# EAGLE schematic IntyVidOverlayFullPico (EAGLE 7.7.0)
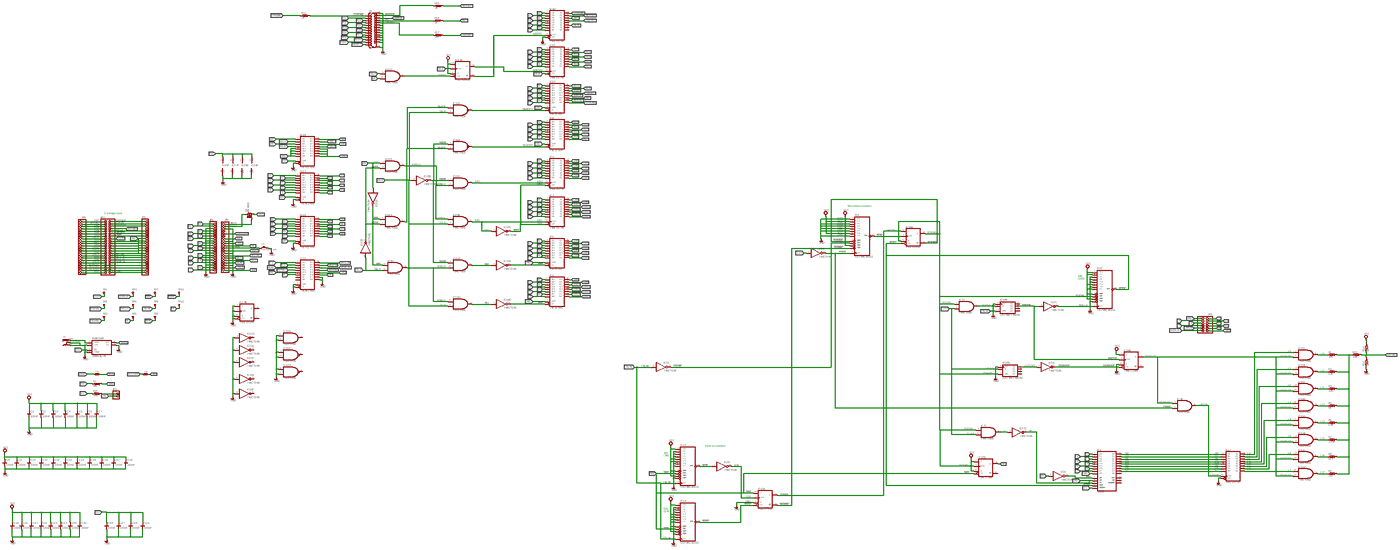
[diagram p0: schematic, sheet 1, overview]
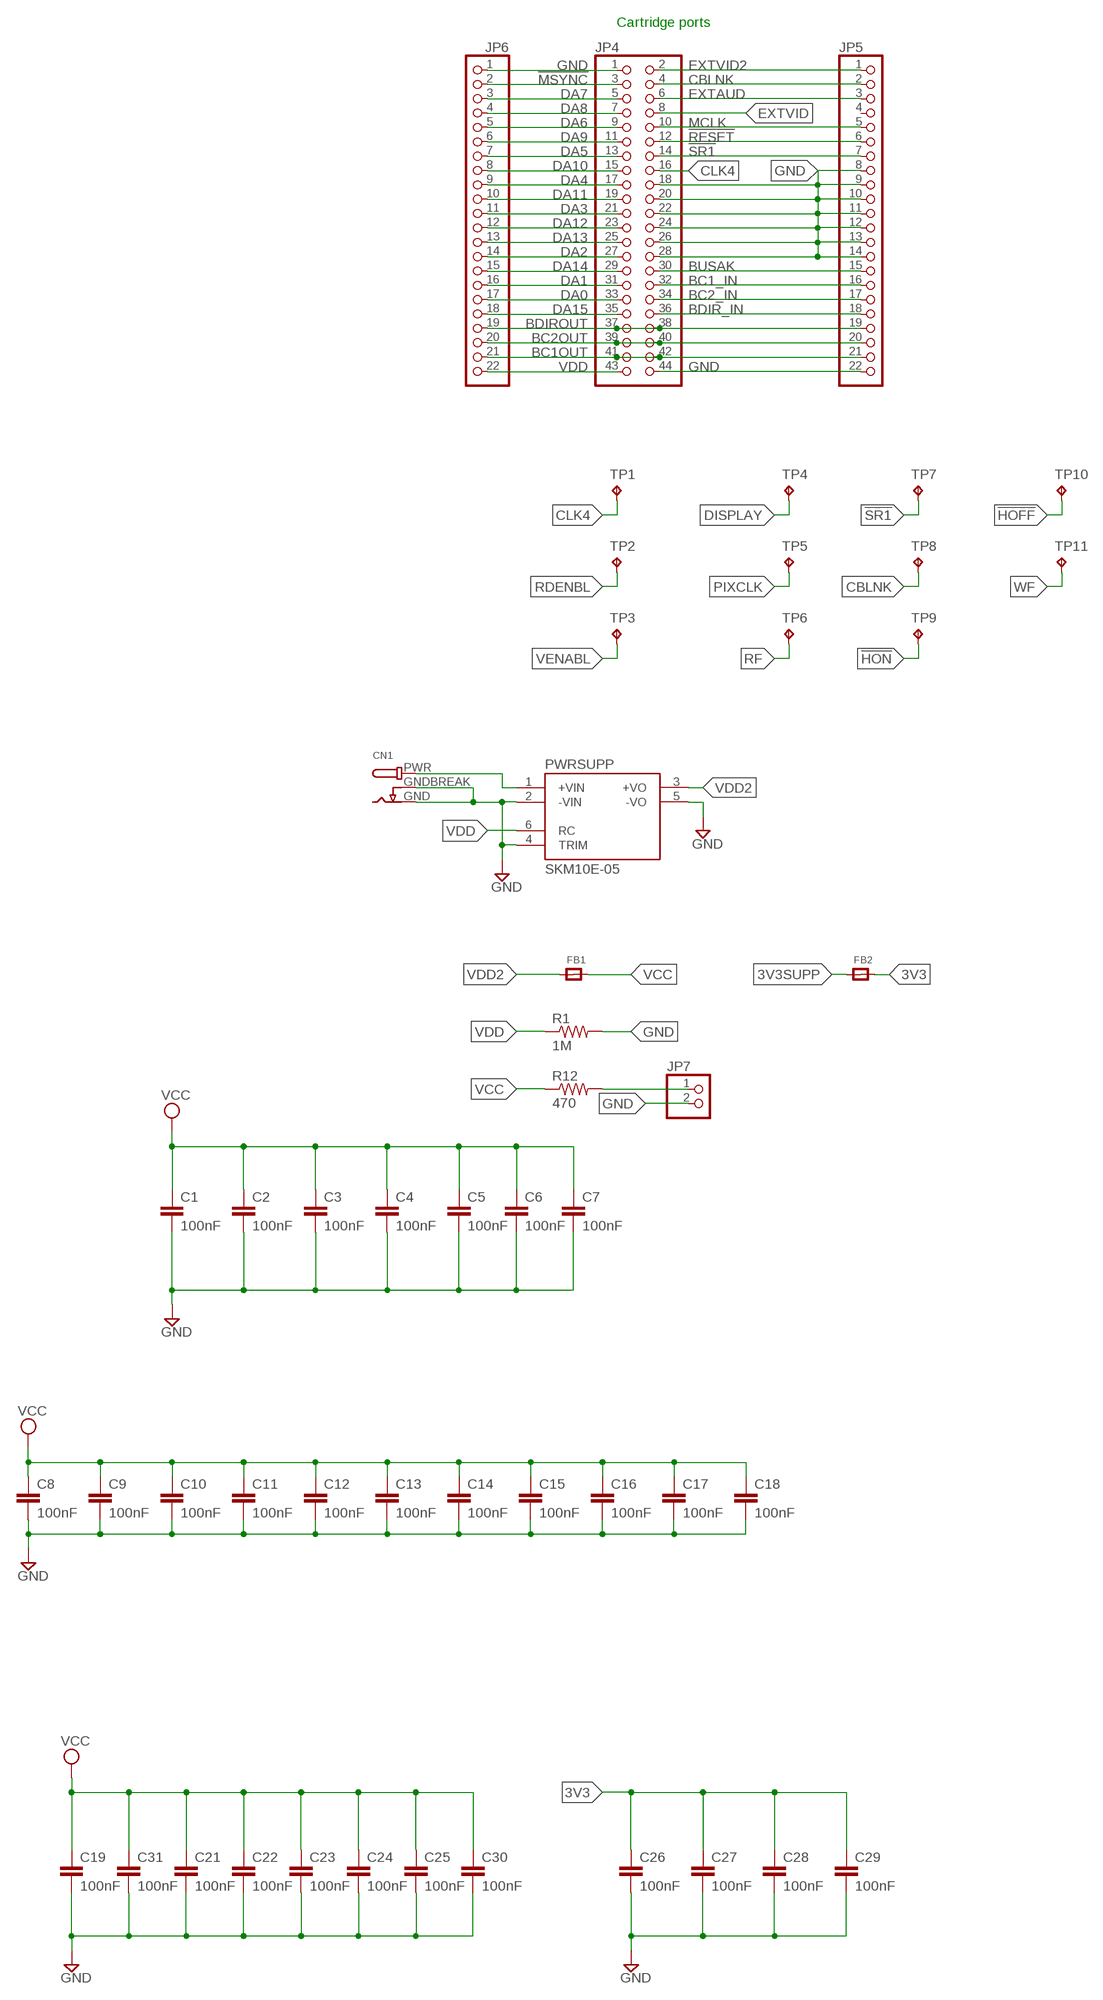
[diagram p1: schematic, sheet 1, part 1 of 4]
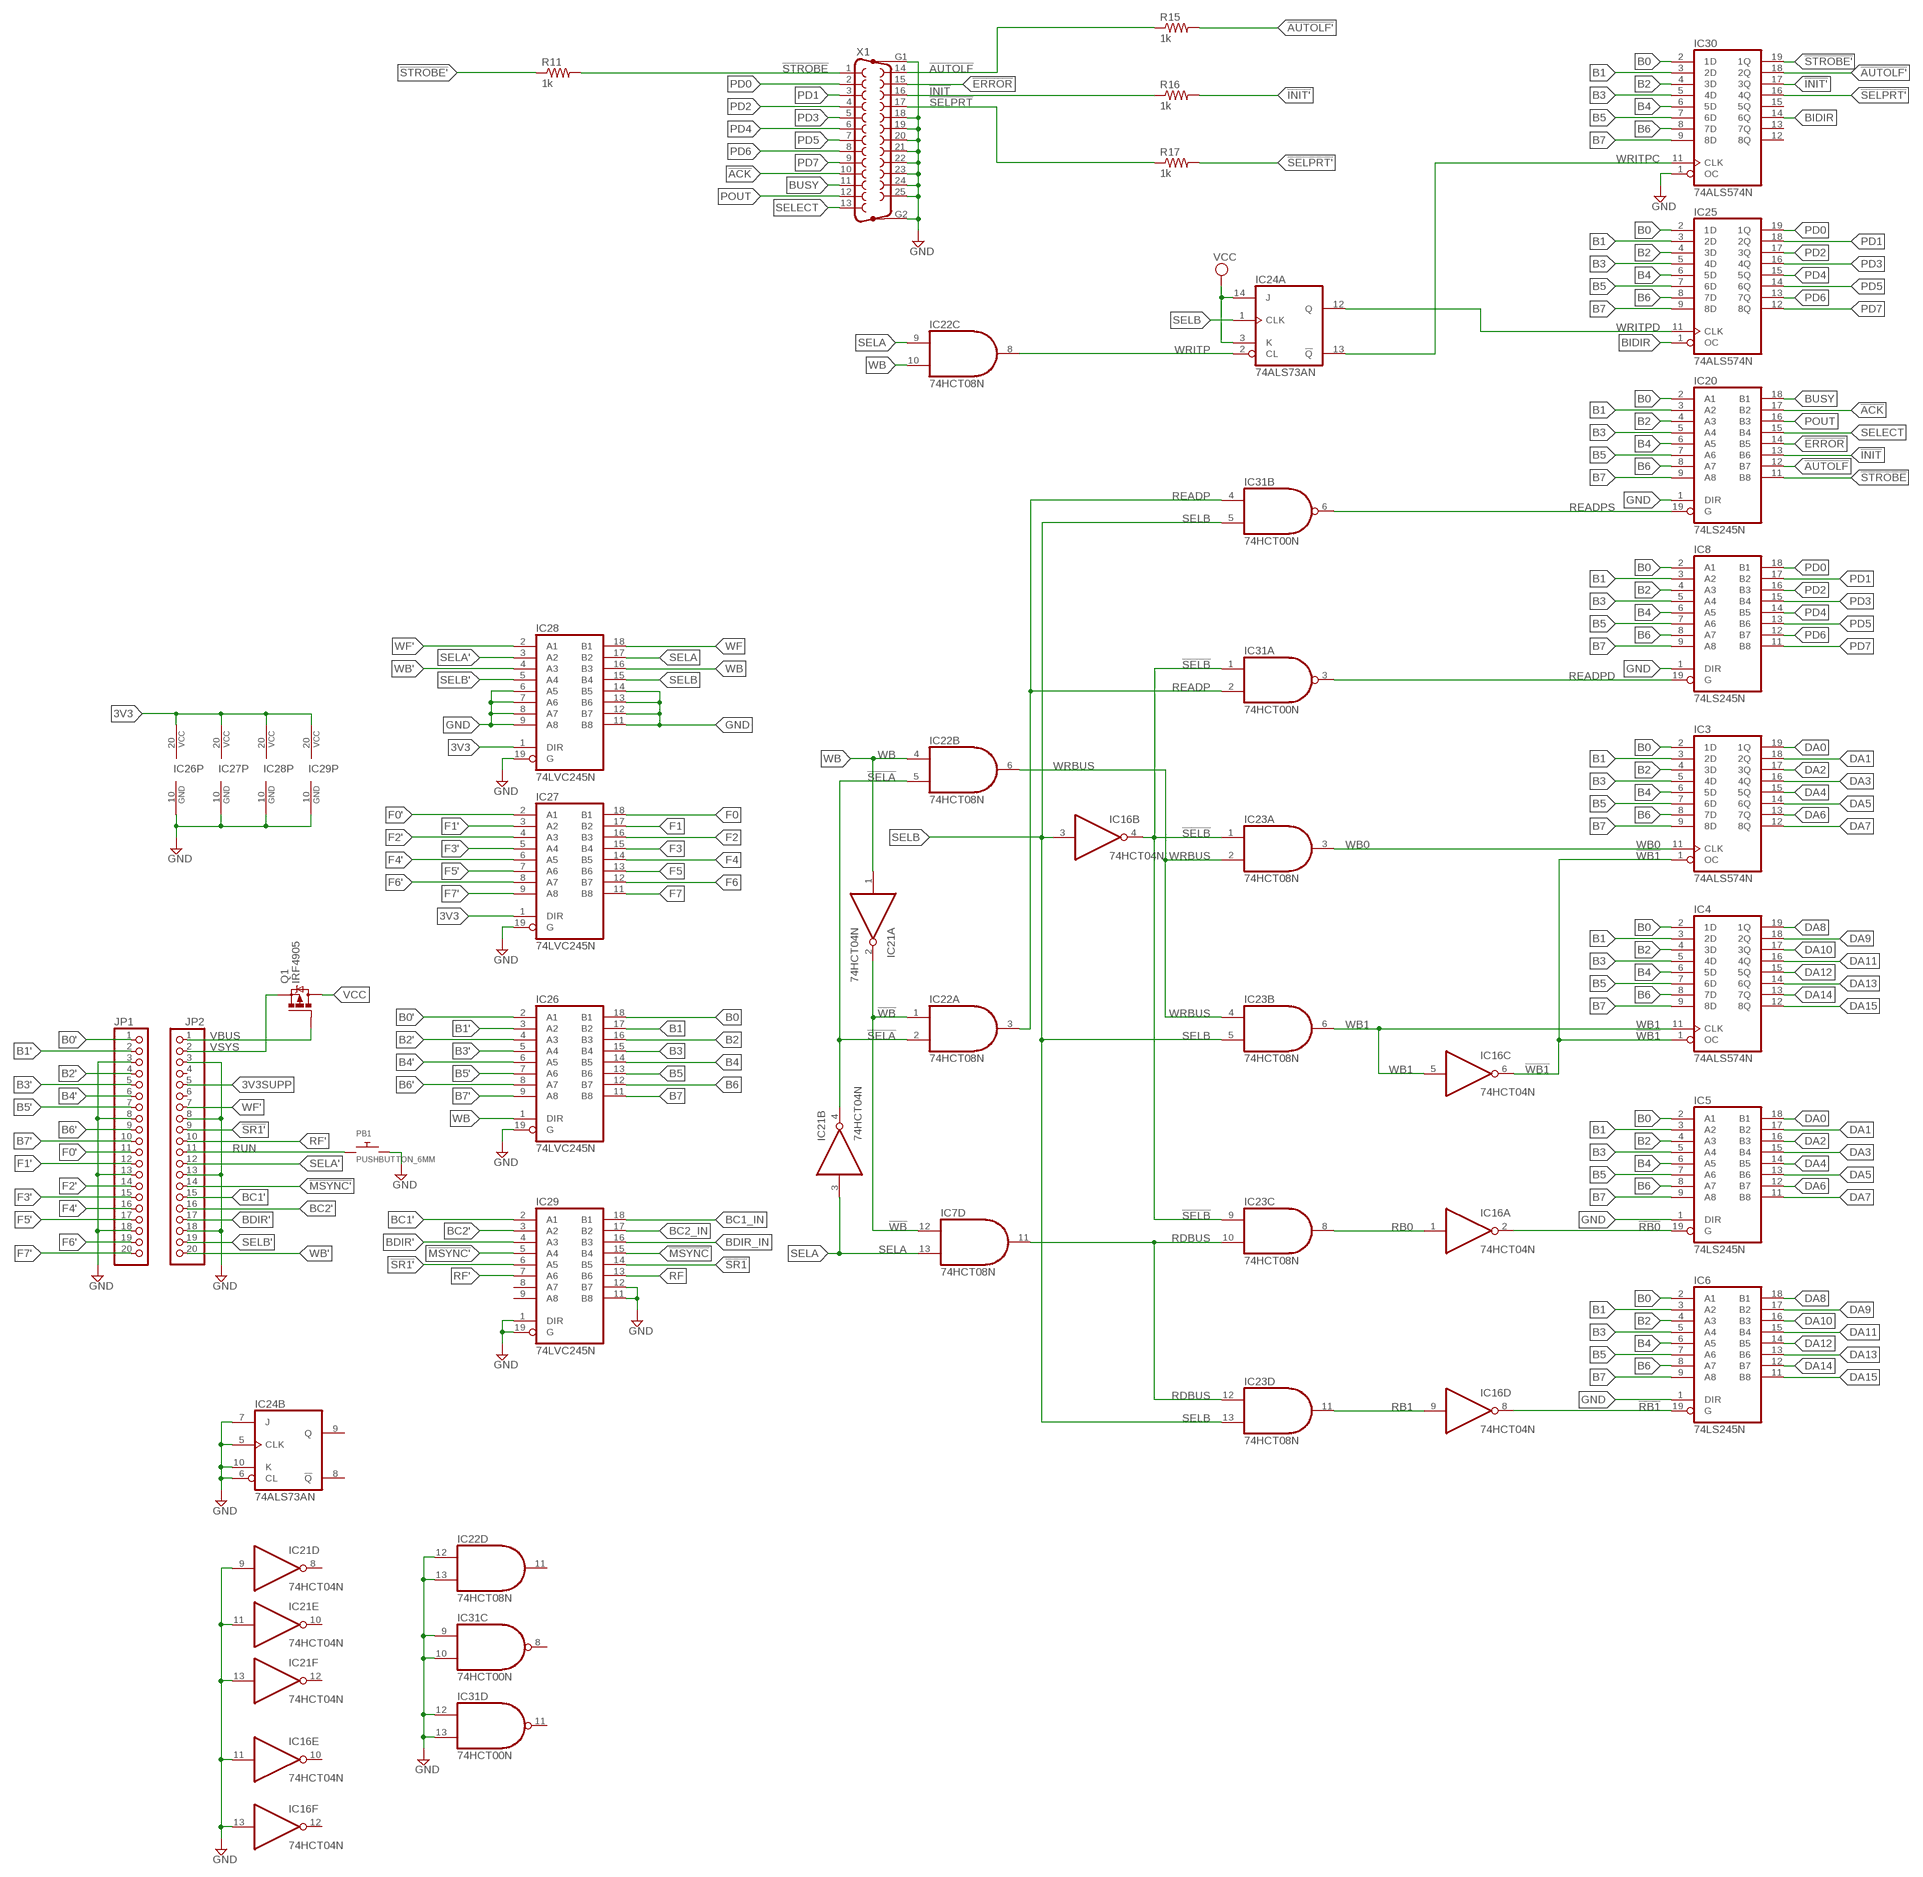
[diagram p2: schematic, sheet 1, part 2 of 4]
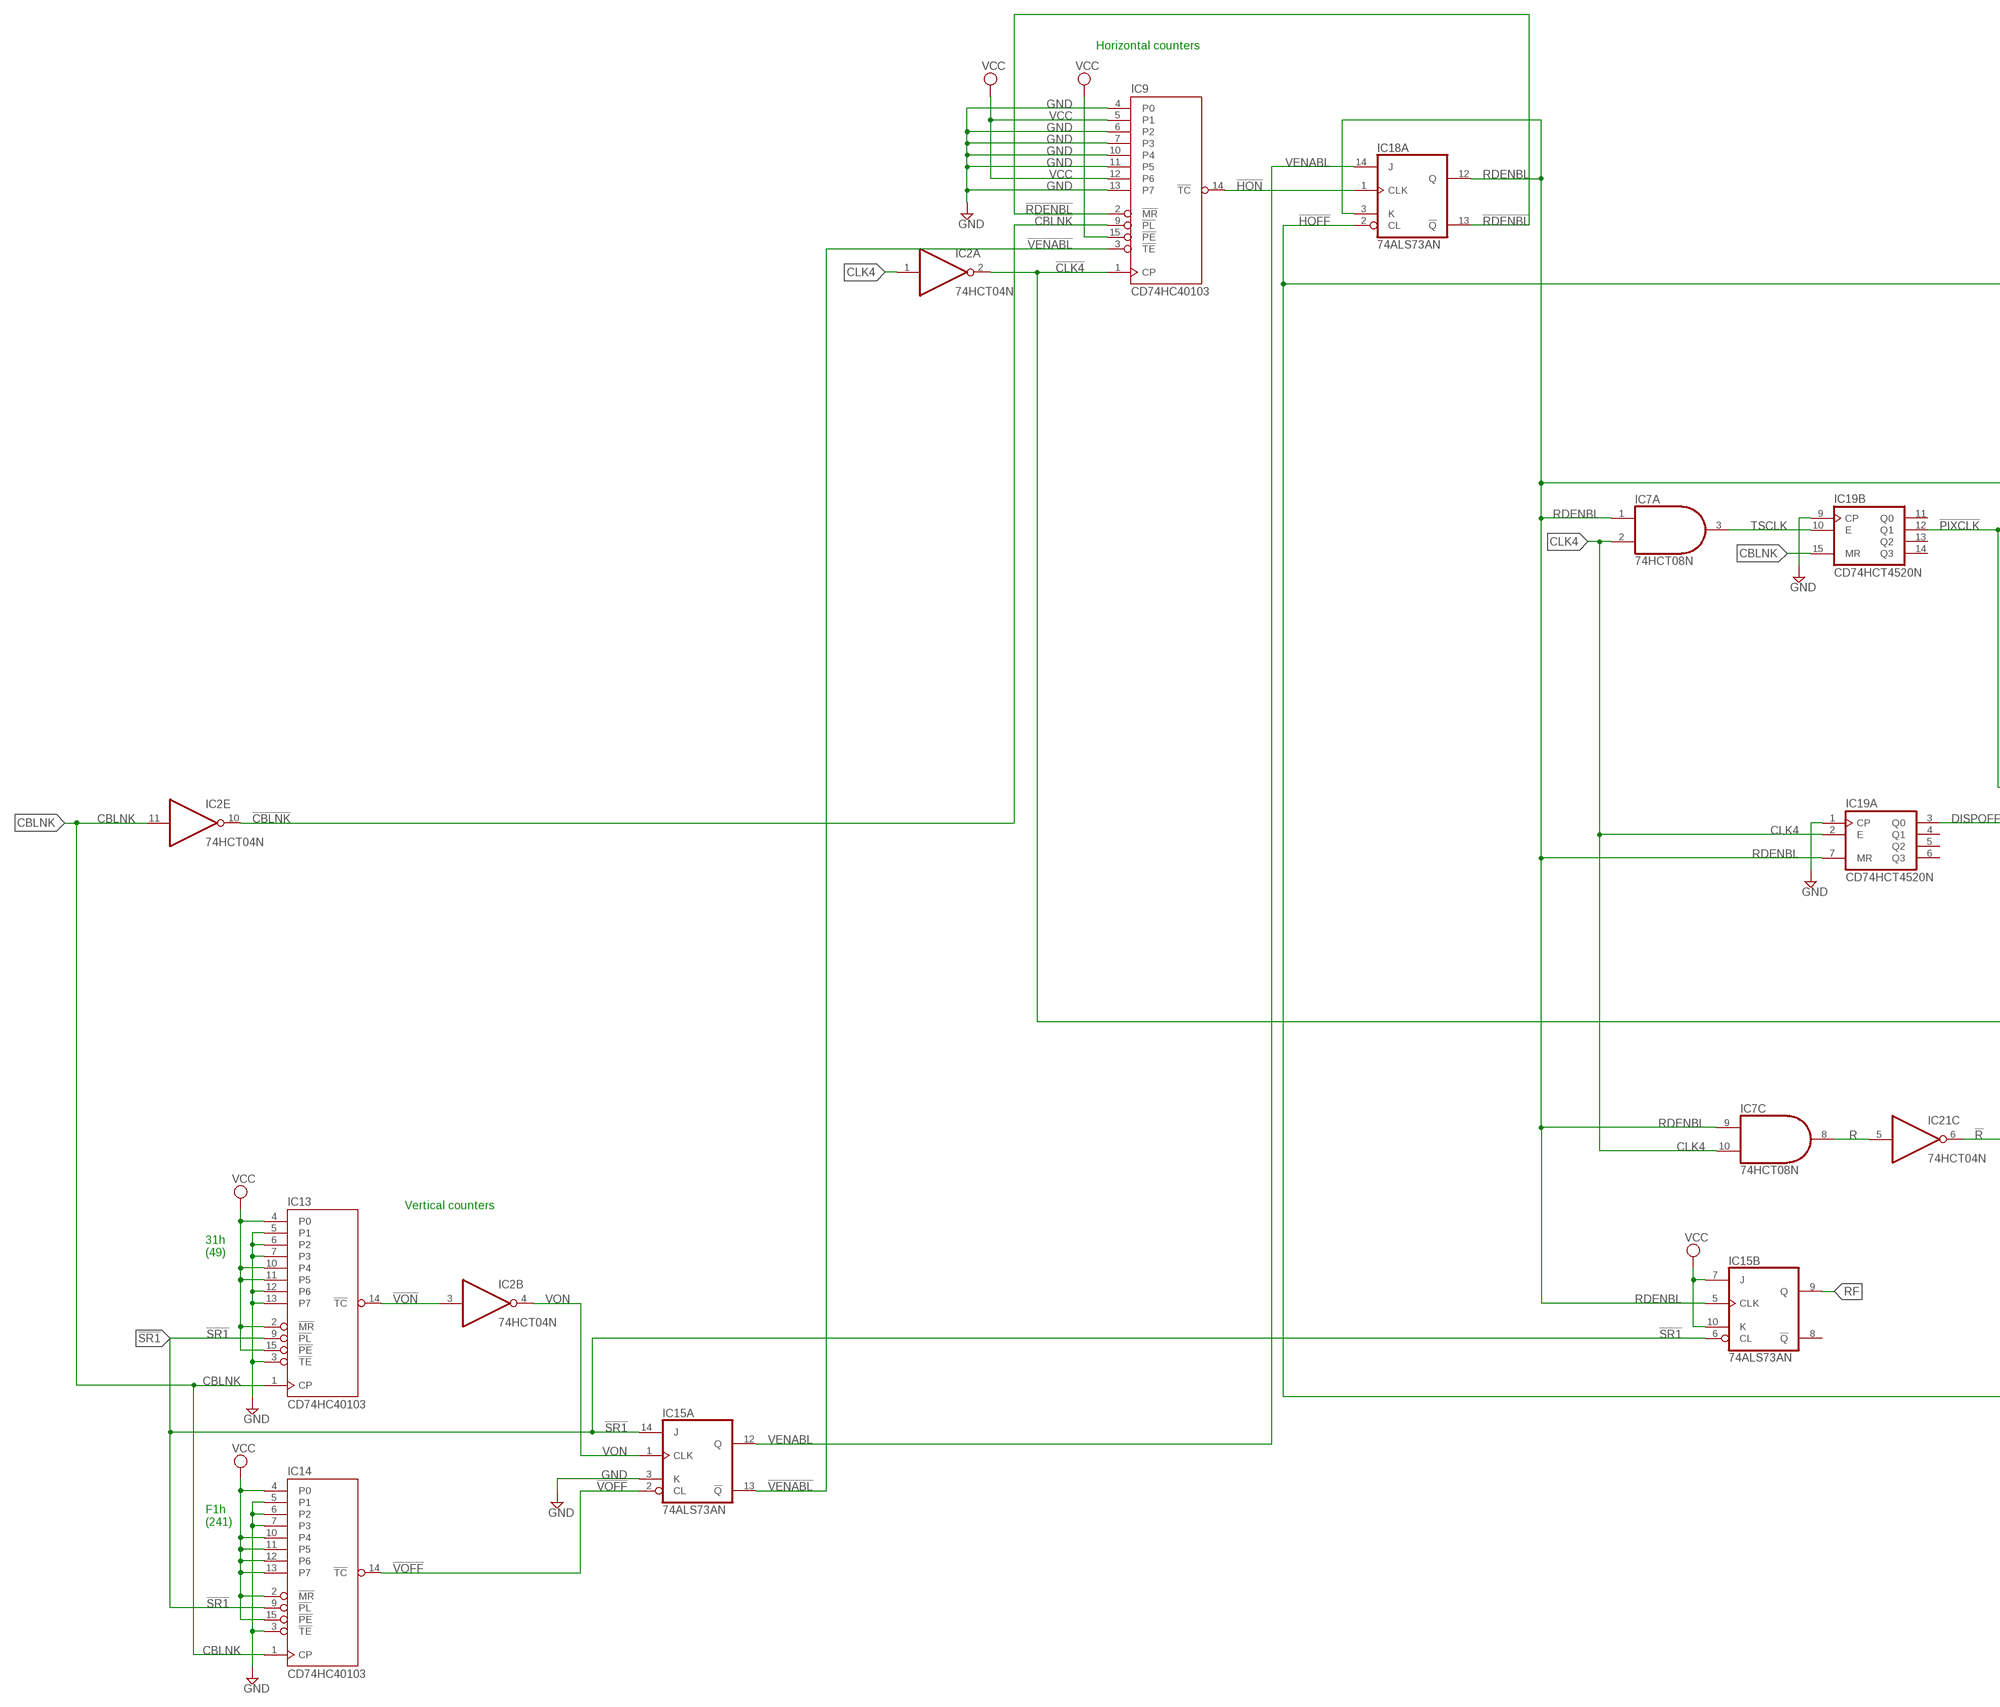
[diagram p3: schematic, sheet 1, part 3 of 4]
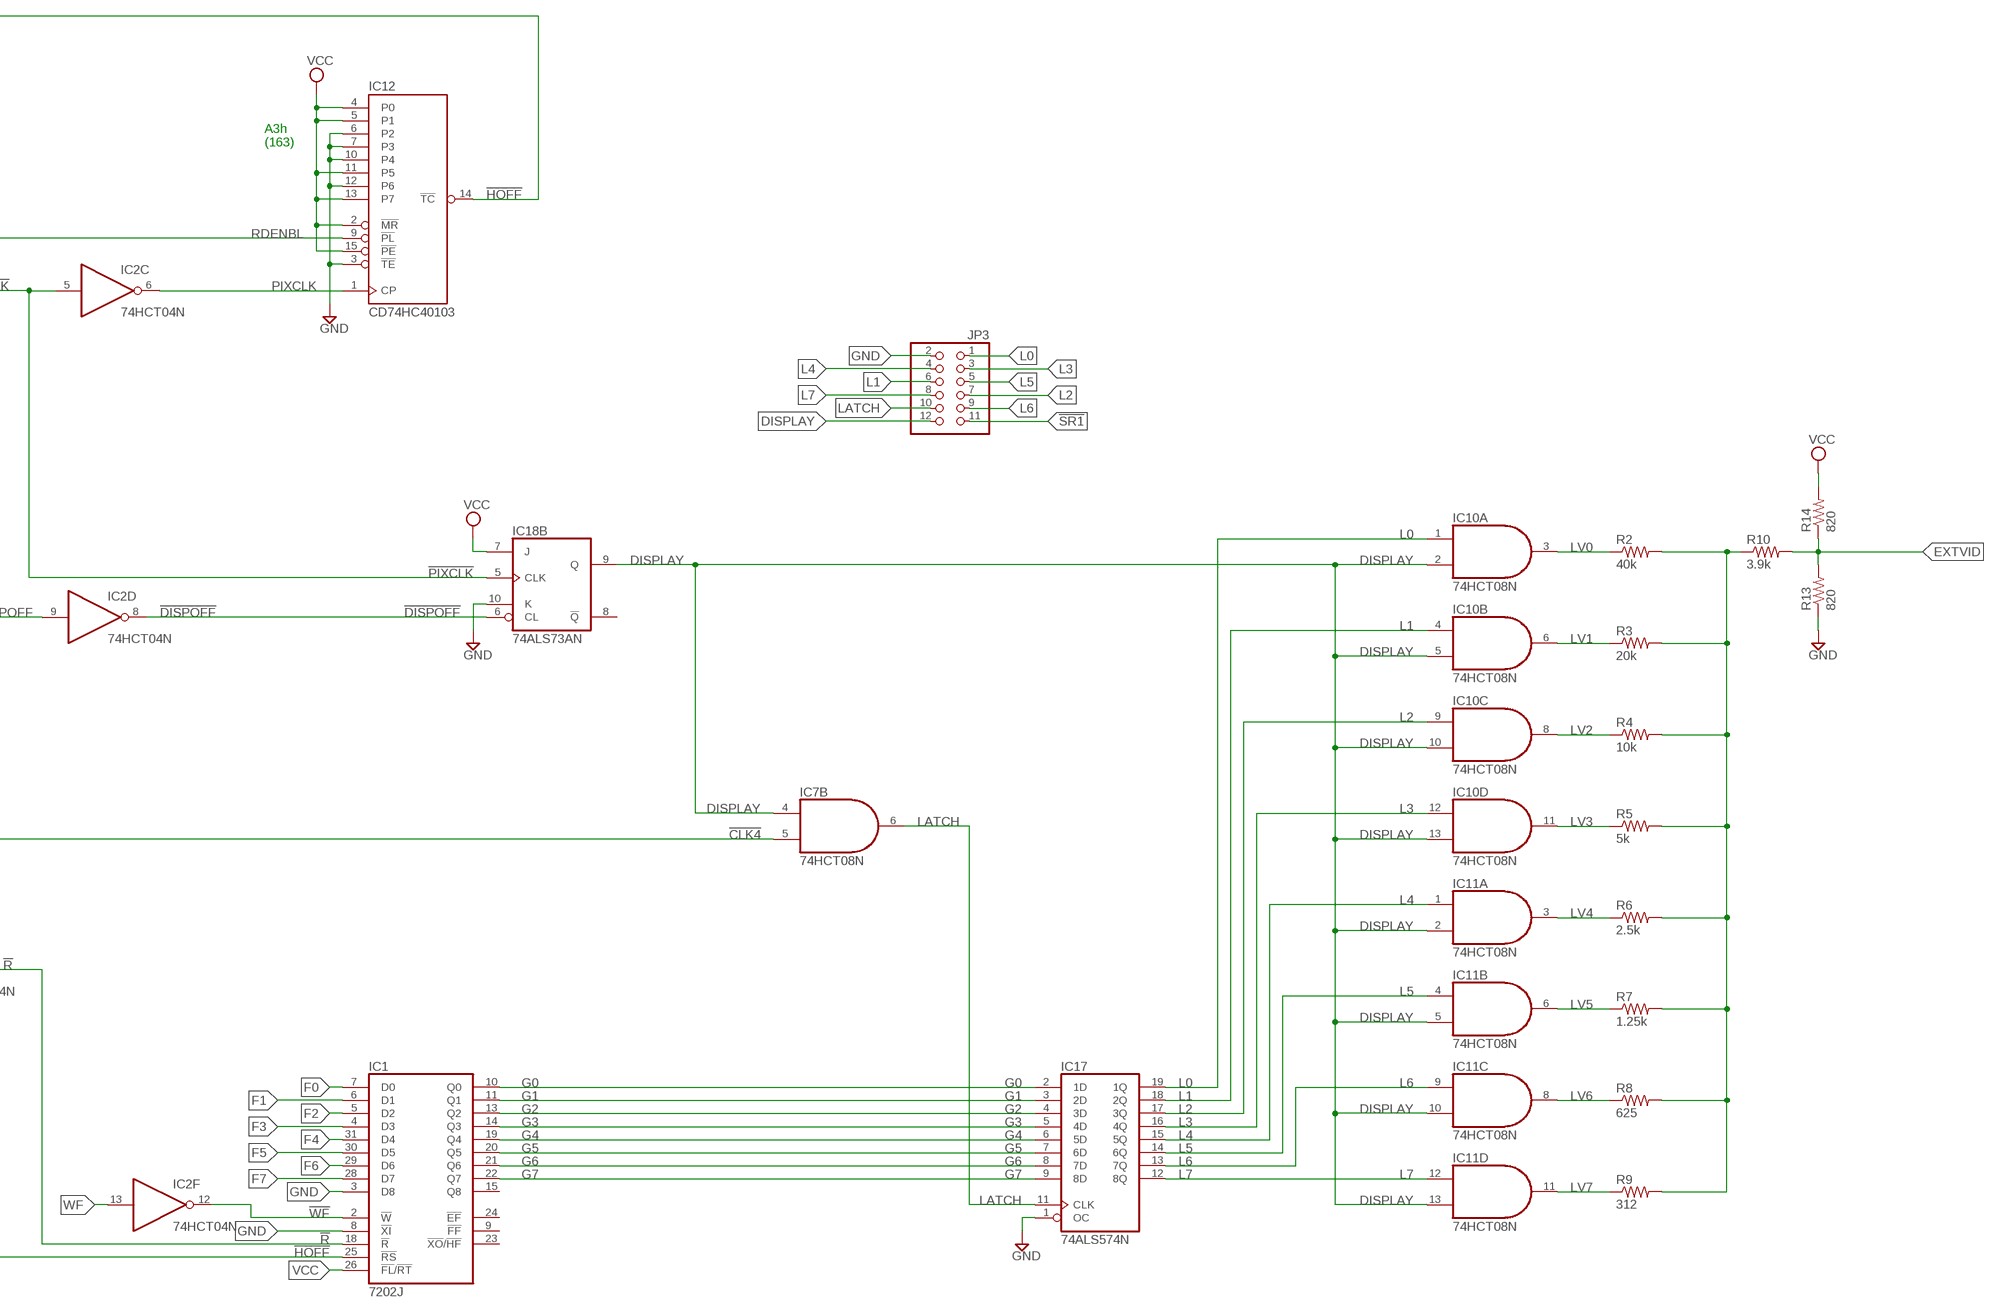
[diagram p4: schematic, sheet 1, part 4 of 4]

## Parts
C1  100nF  CAPPTH  [CAP-PTH-SMALL]
C2  100nF  CAPPTH  [CAP-PTH-SMALL]
C3  100nF  CAPPTH  [CAP-PTH-SMALL]
C4  100nF  CAPPTH  [CAP-PTH-SMALL]
C5  100nF  CAPPTH  [CAP-PTH-SMALL]
C6  100nF  CAPPTH  [CAP-PTH-SMALL]
C7  100nF  CAPPTH  [CAP-PTH-SMALL]
C8  100nF  CAPPTH  [CAP-PTH-SMALL]
C9  100nF  CAPPTH  [CAP-PTH-SMALL]
C10  100nF  CAPPTH  [CAP-PTH-SMALL]
C11  100nF  CAPPTH  [CAP-PTH-SMALL]
C12  100nF  CAPPTH  [CAP-PTH-SMALL]
C13  100nF  CAPPTH  [CAP-PTH-SMALL]
C14  100nF  CAPPTH  [CAP-PTH-SMALL]
C15  100nF  CAPPTH  [CAP-PTH-SMALL]
C16  100nF  CAPPTH  [CAP-PTH-SMALL]
C17  100nF  CAPPTH  [CAP-PTH-SMALL]
C18  100nF  CAPPTH  [CAP-PTH-SMALL]
C19  100nF  CAPPTH  [CAP-PTH-SMALL]
C21  100nF  CAPPTH  [CAP-PTH-SMALL]
C22  100nF  CAPPTH  [CAP-PTH-SMALL]
C23  100nF  CAPPTH  [CAP-PTH-SMALL]
C24  100nF  CAPPTH  [CAP-PTH-SMALL]
C25  100nF  CAPPTH  [CAP-PTH-SMALL]
C26  100nF  CAPPTH  [CAP-PTH-SMALL]
C27  100nF  CAPPTH  [CAP-PTH-SMALL]
C28  100nF  CAPPTH  [CAP-PTH-SMALL]
C29  100nF  CAPPTH  [CAP-PTH-SMALL]
C30  100nF  CAPPTH  [CAP-PTH-SMALL]
C31  100nF  CAPPTH  [CAP-PTH-SMALL]
CN1  DCBARRELPTH  [DCJACK_2MM_PTH]
FB1  FERRITEPTH_0_6  [FERRITE_0_6]
FB2  FERRITEPTH_0_6  [FERRITE_0_6]
IC1  7202J  [PLCC-S32--SOCKET]
IC2  74HCT04N  74LS04N  [DIL14]
IC3  74ALS574N  74AS574N  [DIL20]
IC4  74ALS574N  74AS574N  [DIL20]
IC5  74LS245N  [DIL20]
IC6  74LS245N  [DIL20]
IC7  74HCT08N  74LS08N  [DIL14]
IC8  74LS245N  [DIL20]
IC9  CD74HC40103  [DIL16]
IC10  74HCT08N  74LS08N  [DIL14]
IC11  74HCT08N  74LS08N  [DIL14]
IC12  CD74HC40103  [DIL16]
IC13  CD74HC40103  [DIL16]
IC14  CD74HC40103  [DIL16]
IC15  74ALS73AN  [DIL14]
IC16  74HCT04N  74LS04N  [DIL14]
IC17  74ALS574N  74AS574N  [DIL20]
IC18  74ALS73AN  [DIL14]
IC19  CD74HCT4520N  [DIL16]
IC20  74LS245N  [DIL20]
IC21  74HCT04N  74LS04N  [DIL14]
IC22  74HCT08N  74LS08N  [DIL14]
IC23  74HCT08N  74LS08N  [DIL14]
IC24  74ALS73AN  [DIL14]
IC25  74ALS574N  74AS574N  [DIL20]
IC26  74LVC245N  [DIL20]
IC27  74LVC245N  [DIL20]
IC28  74LVC245N  [DIL20]
IC29  74LVC245N  [DIL20]
IC30  74ALS574N  74AS574N  [DIL20]
IC31  74HCT00N  74LS00N  [DIL14]
JP1  PINHD-1X20OCTAGONAL  [1X20/OCTAGONAL]
JP2  PINHD-1X20OCTAGONAL  [1X20/OCTAGONAL]
JP3  PINHD-2X6  [2X06]
JP4  PINHD-2X22  [2X22]
JP5  PINHD-1X22  [1X22]
JP6  PINHD-1X22  [1X22]
JP7  PINHD-1X2  [1X02]
PB1  PUSHBUTTON_6MM  [PUSHBUTTON_6MM]
PWRSUPP  SKM10E-05  [SKM]
Q1  IRF4905  [TO220BH]
R1  1M  RESISTORPTH-1/2W  [AXIAL-0.5]
R2  40k  RESISTORPTH-1/4W  [AXIAL-0.4]
R3  20k  RESISTORPTH-1/4W  [AXIAL-0.4]
R4  10k  RESISTORPTH-1/4W  [AXIAL-0.4]
R5  5k  RESISTORPTH-1/4W  [AXIAL-0.4]
R6  2.5k  RESISTORPTH-1/4W  [AXIAL-0.4]
R7  1.25k  RESISTORPTH-1/4W  [AXIAL-0.4]
R8  625  RESISTORPTH-1/4W  [AXIAL-0.4]
R9  312  RESISTORPTH-1/4W  [AXIAL-0.4]
R10  3.9k  RESISTORPTH-1/4W  [AXIAL-0.4]
R11  1k  RESISTORPTH-1/4W  [AXIAL-0.4]
R12  470  RESISTORPTH-1/4W  [AXIAL-0.4]
R13  820  RESISTORPTH-1/4W  [AXIAL-0.4]
R14  820  RESISTORPTH-1/4W  [AXIAL-0.4]
R15  1k  RESISTORPTH-1/4W  [AXIAL-0.4]
R16  1k  RESISTORPTH-1/4W  [AXIAL-0.4]
R17  1k  RESISTORPTH-1/4W  [AXIAL-0.4]
TP1  TPB2,54  [B2,54]
TP2  TPB2,54  [B2,54]
TP3  TPB2,54  [B2,54]
TP4  TPB2,54  [B2,54]
TP5  TPB2,54  [B2,54]
TP6  TPB2,54  [B2,54]
TP7  TPB2,54  [B2,54]
TP8  TPB2,54  [B2,54]
TP9  TPB2,54  [B2,54]
TP10  TPB2,54  [B2,54]
TP11  TPB2,54  [B2,54]
X1  F25HP  [F25HP]

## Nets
3V3: C26.1 C27.1 C28.1 C29.1 FB2.P$2 IC26.20(VCC) IC27.1(DIR) IC27.20(VCC) IC28.1(DIR) IC28.20(VCC) IC29.20(VCC)
3V3SUPP: FB2.P$1 JP2.5
!ACK: IC20.17(B2) X1.10
!AUTOLF: IC20.12(B7) R15.P$1 X1.14
!AUTOLF': IC30.18(2Q) R15.P$2
!CBLNK: IC2.10(E:O) IC9.9(!PL)
!CLK4: IC2.2(A:O) IC7.5(B:I1) IC9.1(CP)
!DISPOFF: IC2.8(D:O) IC18.6(B:CL)
!ERROR: IC20.14(B5) X1.15
!HOFF: IC1.25(!RS) IC12.14(!TC) IC18.2(A:CL) TP10.TP
!HON: IC9.14(!TC) IC18.1(A:CLK) TP9.TP
!INIT: IC20.13(B6) R16.P$1 X1.16
!INIT': IC30.17(3Q) R16.P$2
!MSYNC: IC29.15(B4) JP4.3 JP6.2
!MSYNC': IC29.5(A4) JP2.14
!PIXCLK: IC2.5(C:I) IC18.5(B:CLK) IC19.12(B:Q1)
!R: IC1.18(!R) IC21.6(C:O)
!RB0: IC5.19(G) IC16.2(A:O)
!RB1: IC6.19(G) IC16.8(D:O)
!RDENBL: IC9.2(!MR) IC18.13(A:!Q)
!RESET: JP4.12 JP5.6
!SELA: IC21.4(B:O) IC22.2(A:I1) IC22.5(B:I1)
!SELB: IC16.4(B:O) IC23.1(A:I0) IC23.9(C:I0) IC31.1(A:I0)
!SELPRT: R17.P$1 X1.17
!SELPRT': IC30.16(4Q) R17.P$2
!SR1: IC13.9(!PL) IC14.9(!PL) IC15.6(B:CL) IC15.14(A:J) IC29.14(B5) JP3.11 JP4.14 JP5.7 TP7.TP
!SR1': IC29.6(A5) JP2.9
!STROBE: IC20.11(B8) R11.P$2 X1.1
!STROBE': IC30.19(1Q) R11.P$1
!VENABL: IC9.3(!TE) IC15.13(A:!Q)
!VOFF: IC14.14(!TC) IC15.2(A:CL)
!VON: IC2.3(B:I) IC13.14(!TC)
!WB: IC7.12(D:I0) IC21.2(A:O) IC22.1(A:I0)
!WB1: IC3.1(OC) IC4.1(OC) IC16.6(C:O)
!WF: IC1.2(!W) IC2.12(F:O)
B0: IC3.2(1D) IC4.2(1D) IC5.2(A1) IC6.2(A1) IC8.2(A1) IC20.2(A1) IC25.2(1D) IC26.18(B1) IC30.2(1D)
B0': IC26.2(A1) JP1.1
B1: IC3.3(2D) IC4.3(2D) IC5.3(A2) IC6.3(A2) IC8.3(A2) IC20.3(A2) IC25.3(2D) IC26.17(B2) IC30.3(2D)
B1': IC26.3(A2) JP1.2
B2: IC3.4(3D) IC4.4(3D) IC5.4(A3) IC6.4(A3) IC8.4(A3) IC20.4(A3) IC25.4(3D) IC26.16(B3) IC30.4(3D)
B2': IC26.4(A3) JP1.4
B3: IC3.5(4D) IC4.5(4D) IC5.5(A4) IC6.5(A4) IC8.5(A4) IC20.5(A4) IC25.5(4D) IC26.15(B4) IC30.5(4D)
B3': IC26.5(A4) JP1.5
B4: IC3.6(5D) IC4.6(5D) IC5.6(A5) IC6.6(A5) IC8.6(A5) IC20.6(A5) IC25.6(5D) IC26.14(B5) IC30.6(5D)
B4': IC26.6(A5) JP1.6
B5: IC3.7(6D) IC4.7(6D) IC5.7(A6) IC6.7(A6) IC8.7(A6) IC20.7(A6) IC25.7(6D) IC26.13(B6) IC30.7(6D)
B5': IC26.7(A6) JP1.7
B6: IC3.8(7D) IC4.8(7D) IC5.8(A7) IC6.8(A7) IC8.8(A7) IC20.8(A7) IC25.8(7D) IC26.12(B7) IC30.8(7D)
B6': IC26.8(A7) JP1.9
B7: IC3.9(8D) IC4.9(8D) IC5.9(A8) IC6.9(A8) IC8.9(A8) IC20.9(A8) IC25.9(8D) IC26.11(B8) IC30.9(8D)
B7': IC26.9(A8) JP1.10
BC1': IC29.2(A1) JP2.15
BC1_IN: IC29.18(B1) JP4.32 JP5.16
BC1OUT: JP4.41 JP4.42 JP5.21 JP6.21
BC2': IC29.3(A2) JP2.16
BC2_IN: IC29.17(B2) JP4.34 JP5.17
BC2OUT: JP4.39 JP4.40 JP5.20 JP6.20
BDIR': IC29.4(A3) JP2.17
BDIR_IN: IC29.16(B3) JP4.36 JP5.18
BDIROUT: JP4.37 JP4.38 JP5.19 JP6.19
BIDIR: IC25.1(OC) IC30.14(6Q)
BUSAK: JP4.30 JP5.15
BUSY: IC20.18(B1) X1.11
CBLNK: IC2.11(E:I) IC13.1(CP) IC14.1(CP) IC19.15(B:MR) JP4.4 JP5.2 TP8.TP
CLEVEL: R2.P$2 R3.P$2 R4.P$2 R5.P$2 R6.P$2 R7.P$2 R8.P$2 R9.P$2 R10.P$1
CLK4: IC2.1(A:I) IC7.2(A:I1) IC7.10(C:I1) IC19.2(A:E) JP4.16 TP1.TP
DA0: IC3.19(1Q) IC5.18(B1) JP4.33 JP6.17
DA1: IC3.18(2Q) IC5.17(B2) JP4.31 JP6.16
DA2: IC3.17(3Q) IC5.16(B3) JP4.27 JP6.14
DA3: IC3.16(4Q) IC5.15(B4) JP4.21 JP6.11
DA4: IC3.15(5Q) IC5.14(B5) JP4.17 JP6.9
DA5: IC3.14(6Q) IC5.13(B6) JP4.13 JP6.7
DA6: IC3.13(7Q) IC5.12(B7) JP4.9 JP6.5
DA7: IC3.12(8Q) IC5.11(B8) JP4.5 JP6.3
DA8: IC4.19(1Q) IC6.18(B1) JP4.7 JP6.4
DA9: IC4.18(2Q) IC6.17(B2) JP4.11 JP6.6
DA10: IC4.17(3Q) IC6.16(B3) JP4.15 JP6.8
DA11: IC4.16(4Q) IC6.15(B4) JP4.19 JP6.10
DA12: IC4.15(5Q) IC6.14(B5) JP4.23 JP6.12
DA13: IC4.14(6Q) IC6.13(B6) JP4.25 JP6.13
DA14: IC4.13(7Q) IC6.12(B7) JP4.29 JP6.15
DA15: IC4.12(8Q) IC6.11(B8) JP4.35 JP6.18
DISPLAY: IC7.4(B:I0) IC10.2(A:I1) IC10.5(B:I1) IC10.10(C:I1) IC10.13(D:I1) IC11.2(A:I1) IC11.5(B:I1) IC11.10(C:I1) IC11.13(D:I1) IC18.9(B:Q) JP3.12 TP4.TP
DISPOFF: IC2.9(D:I) IC19.3(A:Q0)
EXTAUD: JP4.6 JP5.3
EXTVID: JP4.8 R10.P$2 R13.P$2 R14.P$1
EXTVID2: JP4.2 JP5.1
F0: IC1.7(D0) IC27.18(B1)
F0': IC27.2(A1) JP1.11
F1: IC1.6(D1) IC27.17(B2)
F1': IC27.3(A2) JP1.12
F2: IC1.5(D2) IC27.16(B3)
F2': IC27.4(A3) JP1.14
F3: IC1.4(D3) IC27.15(B4)
F3': IC27.5(A4) JP1.15
F4: IC1.31(D4) IC27.14(B5)
F4': IC27.6(A5) JP1.16
F5: IC1.30(D5) IC27.13(B6)
F5': IC27.7(A6) JP1.17
F6: IC1.29(D6) IC27.12(B7)
F6': IC27.8(A7) JP1.19
F7: IC1.28(D7) IC27.11(B8)
F7': IC27.9(A8) JP1.20
G0: IC1.10(Q0) IC17.2(1D)
G1: IC1.11(Q1) IC17.3(2D)
G2: IC1.13(Q2) IC17.4(3D)
G3: IC1.14(Q3) IC17.5(4D)
G4: IC1.19(Q4) IC17.6(5D)
G5: IC1.20(Q5) IC17.7(6D)
G6: IC1.21(Q6) IC17.8(7D)
G7: IC1.22(Q7) IC17.9(8D)
GND: C1.2 C2.2 C3.2 C4.2 C5.2 C6.2 C7.2 C8.2 C9.2 C10.2 C11.2 C12.2 C13.2 C14.2 C15.2 C16.2 C17.2 C18.2 C19.2 C21.2 C22.2 C23.2 C24.2 C25.2 C26.2 C27.2 C28.2 C29.2 C30.2 C31.2 CN1.GND CN1.GNDBREAK IC1.3(D8) IC1.8(!XI) IC5.1(DIR) IC6.1(DIR) IC8.1(DIR) IC9.4(P0) IC9.6(P2) IC9.7(P3) IC9.10(P4) IC9.11(P5) IC9.13(P7) IC12.3(!TE) IC12.6(P2) IC12.7(P3) IC12.10(P4) IC12.12(P6) IC13.3(!TE) IC13.5(P1) IC13.6(P2) IC13.7(P3) IC13.12(P6) IC13.13(P7) IC14.3(!TE) IC14.5(P1) IC14.6(P2) IC14.7(P3) IC15.3(A:K) IC16.11(E:I) IC16.13(F:I) IC17.1(OC) IC18.10(B:K) IC19.1(A:CP) IC19.9(B:CP) IC20.1(DIR) IC21.9(D:I) IC21.11(E:I) IC21.13(F:I) IC22.12(D:I0) IC22.13(D:I1) IC24.5(B:CLK) IC24.6(B:CL) IC24.7(B:J) IC24.10(B:K) IC26.10(GND) IC26.19(G) IC27.10(GND) IC27.19(G) IC28.6(A5) IC28.7(A6) IC28.8(A7) IC28.9(A8) IC28.10(GND) IC28.11(B8) IC28.12(B7) IC28.13(B6) IC28.14(B5) IC28.19(G) IC29.1(DIR) IC29.10(GND) IC29.11(B8) IC29.12(B7) IC29.19(G) IC30.1(OC) IC31.9(C:I0) IC31.10(C:I1) IC31.12(D:I0) IC31.13(D:I1) JP1.3 JP1.8 JP1.13 JP1.18 JP2.3 JP2.8 JP2.13 JP2.18 JP3.2 JP4.1 JP4.18 JP4.20 JP4.22 JP4.24 JP4.26 JP4.28 JP4.44 JP5.8 JP5.9 JP5.10 JP5.11 JP5.12 JP5.13 JP5.14 JP5.22 JP6.1 JP7.2 PB1.2 PWRSUPP.2(-VIN) PWRSUPP.4(TRIM) PWRSUPP.5(-VO) R1.P$2 R13.P$1 X1.18 X1.19 X1.20 X1.21 X1.22 X1.23 X1.24 X1.25 X1.G1 X1.G2
L0: IC10.1(A:I0) IC17.19(1Q) JP3.1
L1: IC10.4(B:I0) IC17.18(2Q) JP3.6
L2: IC10.9(C:I0) IC17.17(3Q) JP3.7
L3: IC10.12(D:I0) IC17.16(4Q) JP3.3
L4: IC11.1(A:I0) IC17.15(5Q) JP3.4
L5: IC11.4(B:I0) IC17.14(6Q) JP3.5
L6: IC11.9(C:I0) IC17.13(7Q) JP3.9
L7: IC11.12(D:I0) IC17.12(8Q) JP3.8
LATCH: IC7.6(B:O) IC17.11(CLK) JP3.10
LV0: IC10.3(A:O) R2.P$1
LV1: IC10.6(B:O) R3.P$1
LV2: IC10.8(C:O) R4.P$1
LV3: IC10.11(D:O) R5.P$1
LV4: IC11.3(A:O) R6.P$1
LV5: IC11.6(B:O) R7.P$1
LV6: IC11.8(C:O) R8.P$1
LV7: IC11.11(D:O) R9.P$1
MCLK: JP4.10 JP5.5
PD0: IC8.18(B1) IC25.19(1Q) X1.2
PD1: IC8.17(B2) IC25.18(2Q) X1.3
PD2: IC8.16(B3) IC25.17(3Q) X1.4
PD3: IC8.15(B4) IC25.16(4Q) X1.5
PD4: IC8.14(B5) IC25.15(5Q) X1.6
PD5: IC8.13(B6) IC25.14(6Q) X1.7
PD6: IC8.12(B7) IC25.13(7Q) X1.8
PD7: IC8.11(B8) IC25.12(8Q) X1.9
PIXCLK: IC2.6(C:O) IC12.1(CP) TP5.TP
POUT: IC20.16(B3) X1.12
PWR: CN1.PWR PWRSUPP.1(+VIN)
PWRLED: JP7.1 R12.P$2
R: IC7.8(C:O) IC21.5(C:I)
RB0: IC16.1(A:I) IC23.8(C:O)
RB1: IC16.9(D:I) IC23.11(D:O)
RDBUS: IC7.11(D:O) IC23.10(C:I1) IC23.12(D:I0)
RDENBL: IC7.1(A:I0) IC7.9(C:I0) IC12.9(!PL) IC15.5(B:CLK) IC18.3(A:K) IC18.12(A:Q) IC19.7(A:MR) TP2.TP
READP: IC22.3(A:O) IC31.2(A:I1) IC31.4(B:I0)
READPD: IC8.19(G) IC31.3(A:O)
READPS: IC20.19(G) IC31.6(B:O)
RF: IC15.9(B:Q) IC29.13(B6) TP6.TP
RF': IC29.7(A6) JP2.10
RUN: JP2.11 PB1.1
SELA: IC7.13(D:I1) IC21.3(B:I) IC22.9(C:I0) IC28.17(B2)
SELA': IC28.3(A2) JP2.12
SELB: IC16.3(B:I) IC23.5(B:I1) IC23.13(D:I1) IC24.1(A:CLK) IC28.15(B4) IC31.5(B:I1)
SELB': IC28.5(A4) JP2.19
SELECT: IC20.15(B4) X1.13
TSCLK: IC7.3(A:O) IC19.10(B:E)
VBUS: JP2.1 Q1.G
VCC: C1.1 C2.1 C3.1 C4.1 C5.1 C6.1 C7.1 C8.1 C9.1 C10.1 C11.1 C12.1 C13.1 C14.1 C15.1 C16.1 C17.1 C18.1 C19.1 C21.1 C22.1 C23.1 C24.1 C25.1 C30.1 C31.1 FB1.P$2 IC1.26(!FL!/!RT) IC9.5(P1) IC9.12(P6) IC9.15(!PE) IC12.2(!MR) IC12.4(P0) IC12.5(P1) IC12.11(P5) IC12.13(P7) IC12.15(!PE) IC13.2(!MR) IC13.4(P0) IC13.10(P4) IC13.11(P5) IC13.15(!PE) IC14.2(!MR) IC14.4(P0) IC14.10(P4) IC14.11(P5) IC14.12(P6) IC14.13(P7) IC14.15(!PE) IC15.7(B:J) IC15.10(B:K) IC18.7(B:J) IC24.3(A:K) IC24.14(A:J) Q1.D R12.P$1 R14.P$2
VDD: JP4.43 JP6.22 PWRSUPP.6(RC) R1.P$1
VDD2: FB1.P$1 PWRSUPP.3(+VO)
VENABL: IC15.12(A:Q) IC18.14(A:J) TP3.TP
VON: IC2.4(B:O) IC15.1(A:CLK)
VSYS: JP2.2 Q1.S
WB: IC21.1(A:I) IC22.4(B:I0) IC22.10(C:I1) IC26.1(DIR) IC28.16(B3)
WB0: IC3.11(CLK) IC23.3(A:O)
WB1: IC4.11(CLK) IC16.5(C:I) IC23.6(B:O)
WB': IC28.4(A3) JP2.20
WF: IC2.13(F:I) IC28.18(B1) TP11.TP
WF': IC28.2(A1) JP2.7
WRBUS: IC22.6(B:O) IC23.2(A:I1) IC23.4(B:I0)
WRITP: IC22.8(C:O) IC24.2(A:CL)
WRITPC: IC24.13(A:!Q) IC30.11(CLK)
WRITPD: IC24.12(A:Q) IC25.11(CLK)
Unconnected: IC1.9(!FF) IC1.15(Q8) IC1.23(!XO!/!HF) IC1.24(!EF) IC15.8(B:!Q) IC16.10(E:O) IC16.12(F:O) IC18.8(B:!Q) IC19.4(A:Q1) IC19.5(A:Q2) IC19.6(A:Q3) IC19.11(B:Q0) IC19.13(B:Q2) IC19.14(B:Q3) IC21.8(D:O) IC21.10(E:O) IC21.12(F:O) IC22.11(D:O) IC24.8(B:!Q) IC24.9(B:Q) IC29.8(A7) IC29.9(A8) IC30.12(8Q) IC30.13(7Q) IC30.15(5Q) IC31.8(C:O) IC31.11(D:O) JP2.4 JP2.6 JP5.4

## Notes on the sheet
- Horizontal counters
- Cartridge ports
- A3h
  (163)
- Vertical counters
- 31h
  (49)
- F1h
  (241)

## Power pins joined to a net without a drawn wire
GND: IC1.16(GND) IC2.7(P:GND) IC3.10(GND) IC4.10(GND) IC5.10(GND) IC6.10(GND) IC7.7(P:GND) IC8.10(GND) IC9.8(GND) IC10.7(P:GND) IC11.7(P:GND) IC12.8(GND) IC13.8(GND) IC14.8(GND) IC15.11(P:GND) IC16.7(P:GND) IC17.10(GND) IC18.11(P:GND) IC19.8(P:GND) IC20.10(GND) IC21.7(P:GND) IC22.7(P:GND) IC23.7(P:GND) IC24.11(P:GND) IC25.10(GND) IC30.10(GND) IC31.7(P:GND)
VCC: IC1.32(VCC) IC2.14(P:VCC) IC3.20(VCC) IC4.20(VCC) IC5.20(VCC) IC6.20(VCC) IC7.14(P:VCC) IC8.20(VCC) IC9.16(VCC) IC10.14(P:VCC) IC11.14(P:VCC) IC12.16(VCC) IC13.16(VCC) IC14.16(VCC) IC15.4(P:VCC) IC16.14(P:VCC) IC17.20(VCC) IC18.4(P:VCC) IC19.16(P:VCC) IC20.20(VCC) IC21.14(P:VCC) IC22.14(P:VCC) IC23.14(P:VCC) IC24.4(P:VCC) IC25.20(VCC) IC30.20(VCC) IC31.14(P:VCC)

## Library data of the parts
C1-C19 C21-C31 = SparkFun-Capacitors:CAP: Capacitor
CN1 = microbuilder:DCBARREL: DC Barrel Jack DCJACK_1.3MM_PTH - Through Hole 1.3mm Jack (4UConnector: 05536) DCJACK_2MM_PTH - Through Hole 2.0/2.1 Jack (4UConnector: 05537) DCJACK_2MM_SMT - SMT 2.0/2.1mm Jack(4UConnector: 03267)
FB1 FB2 = microbuilder:FERRITE: Ferrite Bead
IC1 = memory-idt:7202: 1k x 9 Asynchronous FIFO
IC2 IC16 IC21 = 74xx-us:74*04: Hex INVERTER
IC3 IC4 IC17 IC25 IC30 = 74xx-us:74*574: 8-bit D type FLIP FLOP bus driver
IC5 IC6 IC8 IC20 IC26-IC29 = 74xx-us:74*245: Octal BUS TRANSCEIVER, 3-state
IC7 IC10 IC11 IC22 IC23 = 74xx-us:74*08: Quad 2-input AND gate
IC9 IC12-IC14 = texas:CD74HC40103: High-Speed CMOS Logic 8-Stage Synchronous Down Counter
IC15 IC18 IC24 = 74xx-us:74*73: Dual J-K FLIP FLOP, clear
IC19 = texas:CD74*4520: Dual syncronous binary UP-COUNTER
IC31 = 74xx-us:74*00: Quad 2-input NAND gate
JP1 JP2 = pinhead:PINHD-1X20: PIN HEADER
JP3 = pinhead:PINHD-2X6: PIN HEADER
JP4 = pinhead:PINHD-2X22: PIN HEADER
JP5 JP6 = pinhead:PINHD-1X22: PIN HEADER
JP7 = pinhead:PINHD-1X2: PIN HEADER
PB1 = microbuilder:PUSHBUTTON_6MM
PWRSUPP = dc-dc:SKM10E-05: MEAN WELL 5V 2A DC-DC Power Converter
Q1 = transistor-power:IRF4905: P-Channel HEXFET® Power MOSFET RDS(on)= 0.02 Ohm, ID = -74A Source: http://www.irf.com/product-info/datasheets/data/irf4905pbf.pdf
R1-R17 = SparkFun-Resistors:RESISTOR: Resistor
TP1-TP11 = testpad:TP: Test pad
X1 = con-subd:F25HP: SUB-D; OC_FARNELL: unknown; OC_NEWARK: unknown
